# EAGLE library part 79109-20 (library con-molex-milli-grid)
RECEPTACAL
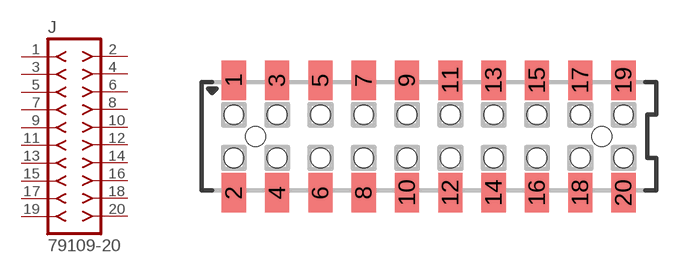
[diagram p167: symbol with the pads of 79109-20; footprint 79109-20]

Designator prefix J

## 79109-20  [79109-20]
1  1  pas
2  2  pas
3  3  pas
4  4  pas
5  5  pas
6  6  pas
7  7  pas
8  8  pas
9  9  pas
10  10  pas
11  11  pas
12  12  pas
13  13  pas
14  14  pas
15  15  pas
16  16  pas
17  17  pas
18  18  pas
19  19  pas
20  20  pas

## Footprint 79109-20 (pad centres in mm)
RECEPTACAL SMD Dual Row, Vertical, Pass-Thru
smd 1.12 x 1.83: 1 -9,2.6; 2 -9,-2.6; 3 -7,2.6; 4 -7,-2.6; 5 -5,2.6; 6 -5,-2.6; 7 -3,2.6; 8 -3,-2.6; 9 -1,2.6; 10 -1,-2.6; 11 1,2.6; 12 1,-2.6; 13 3,2.6; 14 3,-2.6; 15 5,2.6; 16 5,-2.6; 17 7,2.6; 18 7,-2.6; 19 9,2.6; 20 9,-2.6
hole 0.914 at -8,0
hole 0.914 at -9,1
hole 0.914 at -9,-1
hole 0.914 at -7,-1
hole 0.914 at -7,1
hole 0.914 at -5,-1
hole 0.914 at -5,1
hole 0.914 at 8,0
hole 0.914 at -3,1
hole 0.914 at -3,-1
hole 0.914 at -1,1
hole 0.914 at -1,-1
hole 0.914 at 1,1
hole 0.914 at 1,-1
hole 0.914 at 3,1
hole 0.914 at 3,-1
hole 0.914 at 5,-1
hole 0.914 at 5,1
hole 0.914 at 7,1
hole 0.914 at 7,-1
hole 0.914 at 9,1
hole 0.914 at 9,-1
